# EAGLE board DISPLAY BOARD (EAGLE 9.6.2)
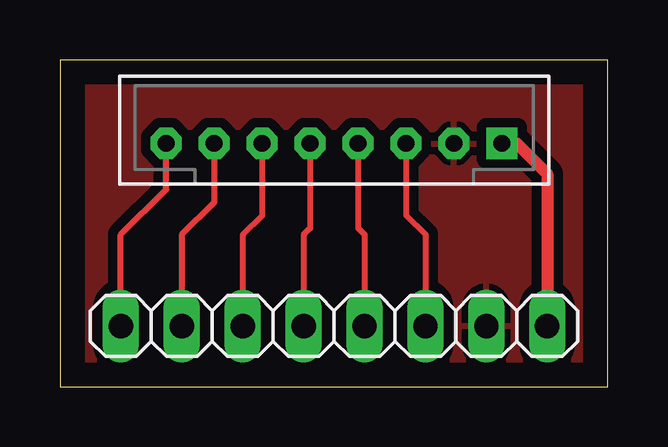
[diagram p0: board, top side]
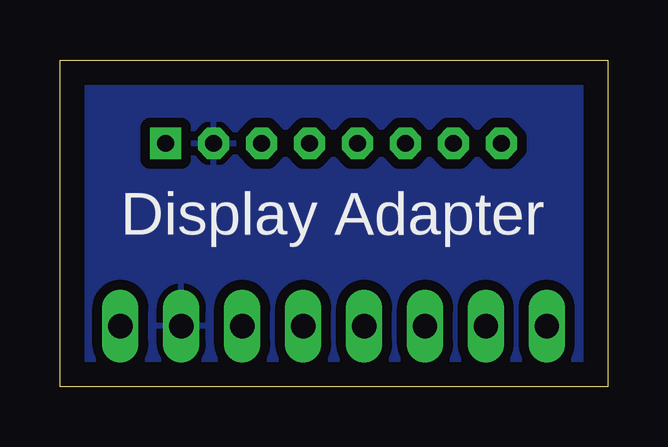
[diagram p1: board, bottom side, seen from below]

Size 22.84 x 13.64 mm. Coordinates in mm from the lower left corner, seen from the top.
Outline: 0,0 22.84,0 22.84,13.64 0,13.64 0,0
Copper layers (1*16): Top 0.035mm / dielectric 1.5mm / Bottom 0.035mm
Design rules "default": minimum track width 6mil, minimum drill 0.35mm, track to track 6mil, track to pad 6mil, pad to pad 6mil, via to via 6mil, smd to smd 6mil, copper to edge 40mil, drill to drill 6mil, minimum pad ring 10mil, minimum via ring 8mil, stop-mask expansion 4mil, vias tented up to drill 0mil, thermal gap 10mil

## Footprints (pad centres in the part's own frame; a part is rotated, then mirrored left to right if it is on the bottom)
1X08 = drill 1.016 long: 1 -8.89,0; 2 -6.35,0; 3 -3.81,0; 4 -1.27,0; 5 1.27,0; 6 3.81,0; 7 6.35,0; 8 8.89,0
B8B-PH-K-S = drill 0.7 pad 1.3 square: 1 7,0 | drill 0.7 pad 1.3 octagon: 2 5,0; 3 3,0; 4 1,0; 5 -1,0; 6 -3,0; 7 -5,0; 8 -7,0

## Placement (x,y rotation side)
JP1  [1X08]  11.43,2.54 0 top
X1  B8B-PH-K-S  [B8B-PH-K-S]  11.43,10.16 0 top

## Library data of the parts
JP1 = pinhead
X1 = con-JSTPH

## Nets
3,3V: JP1.8 X1.1
BUSY: JP1.1 X1.8
CS: JP1.4 X1.5
DC: JP1.3 X1.6
GND: JP1.7 X1.2
RES: JP1.2 X1.7
SCK: JP1.5 X1.4
SDI: JP1.6 X1.3

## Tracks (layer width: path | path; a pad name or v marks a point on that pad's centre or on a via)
3,3V
  Top 0.508: X1.1 19.05,10.16 20.32,8.89 JP1.8
BUSY
  Top 0.254: X1.8 4.43,8.24 2.54,6.35 JP1.1
CS
  Top 0.254: X1.5 10.43,6.62 10.16,6.35 JP1.4
DC
  Top 0.254: X1.6 8.43,7.16 7.62,6.35 JP1.3
GND
  pour Top (isolate 0.406): 0,13.97 22.86,13.97 22.86,0 0,0
  pour Bottom (isolate 0.406): 0,13.97 22.86,13.97 22.86,0 0,0
RES
  Top 0.254: X1.7 6.43,7.7 5.08,6.35 JP1.2
SCK
  Top 0.254: X1.4 12.43,6.62 12.7,6.35 JP1.5
SDI
  Top 0.254: JP1.6 15.24,6.35 14.43,7.16 X1.3

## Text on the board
bPlace: Display Adapter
